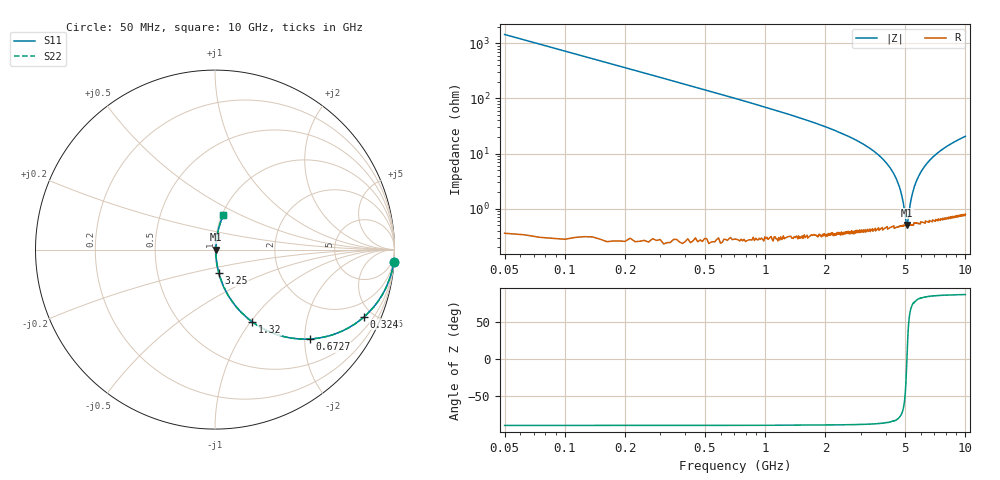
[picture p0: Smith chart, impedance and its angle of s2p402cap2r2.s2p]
! AVX Thin Film Operation		Date: January 2010
! Description: Accu-P® Series, Thin Film, SMD, RF Capacitor
! Part Number: 04021J2R2ABS
! 50 MHz  -  10 GHz
! Serial Measurements
#	MHZ	S	MA	R	50
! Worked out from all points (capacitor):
!   800 points, 50 MHz to 10 GHz, reference 50 ohm
!   read as one part in series: C = 2.2 pF near 99.81 MHz
!   lowest |Z| = 504 mohm at 5.106 GHz (marker M1)
!   series resonance near 5.103 GHz, so ESL is about 440 pH
!   S11 on the Smith chart (normalised r, x): 50 MHz: 1, -29; 324 MHz: 1.00, -4.45; 672.7 MHz: 1.01, -2.11; 1.32 GHz: 1.01, -1.02; 3.25 GHz: 1.01, -0.27; 10 GHz: 1.02, +0.41
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50  0.998 -4.0  0.069 86.0  0.069 86.0  0.998 -4.0
174.531  0.972 -13.6  0.235 76.4  0.235 76.4  0.972 -13.6
323.967  0.912 -24.2  0.41 65.7  0.41 65.7  0.912 -24.2
672.653  0.725 -43.3  0.686 46.5  0.686 46.5  0.725 -43.3
971.527  0.582 -54.2  0.811 35.6  0.811 35.6  0.582 -54.2
1320.213  0.454 -62.7  0.888 27.0  0.888 27.0  0.454 -62.7
1718.711  0.349 -69.1  0.934 20.4  0.934 20.4  0.349 -69.1
3250.438  0.131 -80.8  0.987 7.5  0.987 7.5  0.131 -80.8
3374.969  0.119 -81.2  0.989 6.8  0.989 6.8  0.119 -81.2
4034.981  0.067 -82.4  0.993 3.8  0.993 3.8  0.067 -82.4
4495.745  0.036 -80.5  0.995 2.1  0.995 2.1  0.036 -80.5
4819.524  0.017 -72.3  0.995 0.9  0.995 0.9  0.017 -72.3
5031.227  0.00637 -38.3  0.995 0.2  0.995 0.2  0.00637 -38.3
5105.945  0.00503 2.2  0.995 -0.0  0.995 -0.0  0.00503 2.2
5155.757  0.00584 29.9  0.995 -0.2  0.995 -0.2  0.00584 29.9
5305.194  0.012 64.3  0.995 -0.6  0.995 -0.6  0.012 64.3
5404.819  0.017 71.4  0.995 -0.9  0.995 -0.9  0.017 71.4
5666.333  0.03 78.1  0.994 -1.7  0.994 -1.7  0.03 78.1
6089.737  0.05 80.8  0.993 -2.9  0.993 -2.9  0.05 80.8
6687.484  0.077 81.2  0.991 -4.4  0.991 -4.4  0.077 81.2
8343.742  0.143 79.1  0.983 -8.2  0.983 -8.2  0.143 79.1
10000  0.2 76.3  0.972 -11.5  0.972 -11.5  0.2 76.3
